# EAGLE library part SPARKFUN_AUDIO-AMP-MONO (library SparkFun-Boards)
SparkFun Mono Audio Amp Breakout- TPA2005D1 This tiny audio amplifier is based on the Texas Instruments TPA2005D1. Its efficient class-D operation means low heat and long battery life. It can drive an 8-Ohm speaker at up to 1.4 Watts SparkFun Products: Mono Audio Amp Breakout
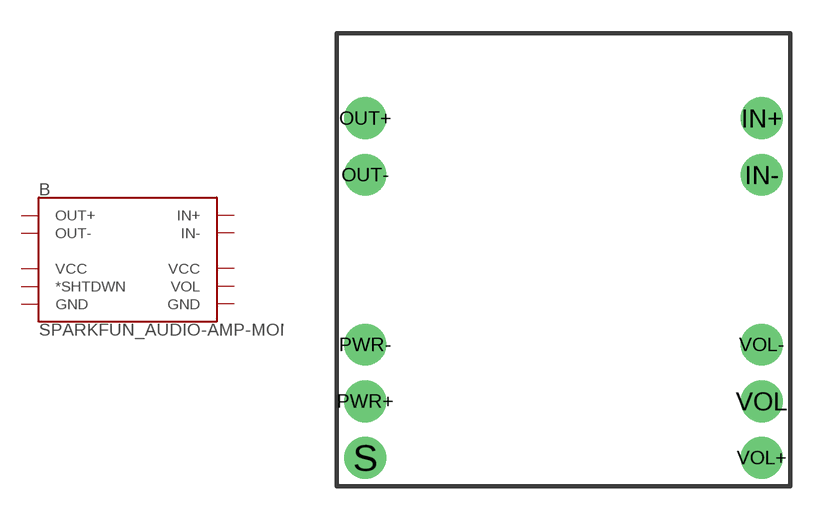
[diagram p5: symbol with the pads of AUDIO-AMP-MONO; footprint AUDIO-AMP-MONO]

Designator prefix B

## SPARKFUN_AUDIO-AMP-MONODIP  [AUDIO-AMP-MONO]
IN+  IN+
IN-  IN-
OUT+  OUT+
OUT-  OUT-
PWR+  VCC
PWR-  GND
S  *SHTDWN
VOL  VOL
VOL+  VCC
VOL-  GND

## Footprint AUDIO-AMP-MONO (pad centres in mm)
Audio Amp Mono PCB Specifications: Pin count: 10 Pin pitch: 0.1" Area:0.8x0.8 in Example device(s): Audio Amp Mono
drill 1.016 pad 1.88: IN+ 8.89,6.35; IN- 8.89,3.81; OUT+ -8.89,6.35; OUT- -8.89,3.81; PWR+ -8.89,-6.35; PWR- -8.89,-3.81; S -8.89,-8.89; VOL 8.89,-6.35; VOL+ 8.89,-8.89; VOL- 8.89,-3.81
